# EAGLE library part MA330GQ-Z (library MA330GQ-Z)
14-Bit Digital Contactless Angle Sensor with ABZ & UVW Incremental Outputs 16-Pin QFN T/R - Tape and Reel Source: Datasheet
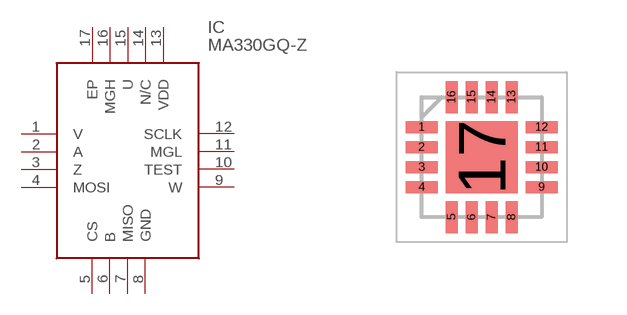
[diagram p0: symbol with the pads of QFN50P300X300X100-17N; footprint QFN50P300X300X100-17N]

Designator prefix IC

## MA330GQ-Z (Description: 14-Bit Digital Contactless Angle Sensor with ABZ & UVW Incremental Outputs 16-Pin QFN T/R - Tape and Reel; Height: 1mm; Manufacturer_Name: Monolithic Power Systems (MPS); Manufacturer_Part_Number: MA330GQ-Z; Mouser_Part_Number: 946-MA330GQ-Z; Mouser_Price-Stock: https://www.mouser.co.uk/ProductDetail/Monolithic-Power-Systems-MPS/MA330GQ-Z?qs=Zz7%252BYVVL6bHPpcm%252B14Y%2FHg%3D%3D)  [QFN50P300X300X100-17N]
1  V
2  A
3  Z
4  MOSI
5  CS
6  B
7  MISO
8  GND
9  W
10  TEST
11  MGL
12  SCLK
13  VDD
14  N/C  nc
15  U
16  MGH
17  EP

## Footprint QFN50P300X300X100-17N (pad centres in mm)
QFN-16 (3mmx3mm)
smd 0.8 x 0.3: 1 -1.5,0.75; 2 -1.5,0.25; 3 -1.5,-0.25; 4 -1.5,-0.75; 9 1.5,-0.75; 10 1.5,-0.25; 11 1.5,0.25; 12 1.5,0.75
smd 0.3 x 0.8: 5 -0.75,-1.5; 6 -0.25,-1.5; 7 0.25,-1.5; 8 0.75,-1.5; 13 0.75,1.5; 14 0.25,1.5; 15 -0.25,1.5; 16 -0.75,1.5
smd 1.8 x 1.8: 17 0,0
